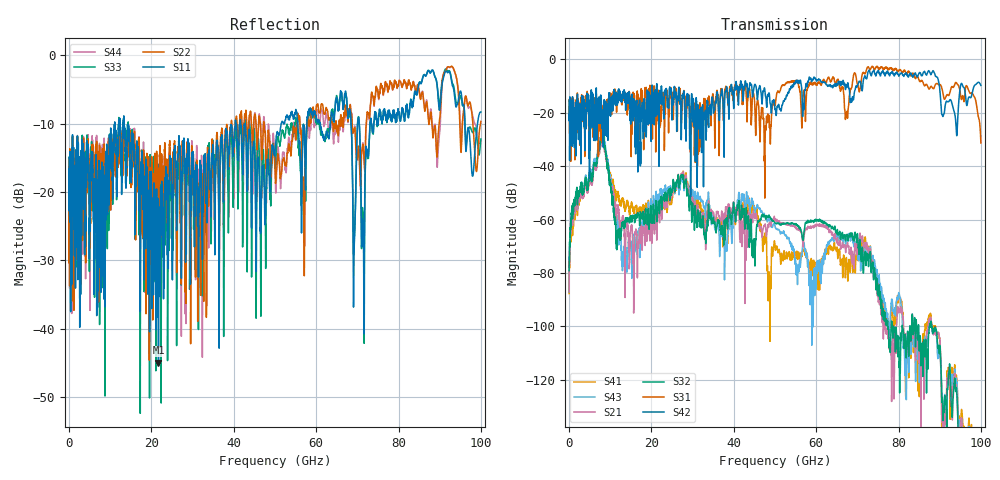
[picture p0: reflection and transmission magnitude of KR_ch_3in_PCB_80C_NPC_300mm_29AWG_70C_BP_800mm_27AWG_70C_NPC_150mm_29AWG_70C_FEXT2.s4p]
# Hz S RI R 45
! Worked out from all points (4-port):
!   4000 points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, 25 MHz to 100 GHz, reference 45 ohm
!   strongest paths, dB at 25 MHz, 25.02 GHz, 50.02 GHz, 75.03 GHz, 100 GHz:
!     S42: -20.7, -20.7, -18.8, -4.2, -9.7
!     S31: -20.6, -14.0, -17.0, -3.0, -31.3
!     S32: -79.1, -49.3, -61.3, -85.7, -155.2
!     S21: -86.9, -50.5, -60.1, -87.3, -157.5
!     S43: -87.1, -48.7, -62.6, -81.8, -149.2
!     S41: -87.7, -52.4, -69.9, -83.4, -149.2
!   lowest |S11| = -45.0 dB at 21.73 GHz (marker M1), VSWR 1.01, Z = 44.8 + j0.478 ohm
!   |S11| at or under -10 dB: start of sweep to 11.1 GHz; 13.4 GHz to 40.37 GHz (26.97 GHz wide, 100 % of centre); 42.78 GHz to 51.51 GHz (8.731 GHz wide, 18.5 % of centre)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
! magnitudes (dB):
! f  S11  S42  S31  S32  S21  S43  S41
! 25 MHz  -16.6  -20.7  -20.6  -79.1  -86.9  -87.1  -87.7
! 8 GHz  -16.5  -25.6  -24.5  -27.7  -29.6  -26.5  -28.3
! 13.22 GHz  -9.5  -12.1  -13.5  -61.6  -60.0  -72.9  -53.3
! 21.73 GHz  -45.0  -14.0  -18.2  -53.1  -56.2  -50.5  -53.9
! 27.5 GHz  -18.5  -13.4  -19.0  -43.2  -42.5  -44.5  -42.6
! 76.92 GHz  -9.4  -5.0  -2.8  -98.9  -102.3  -93.4  -96.0
! 100 GHz  -8.3  -9.7  -31.3  -155.2  -157.5  -149.2  -149.2
